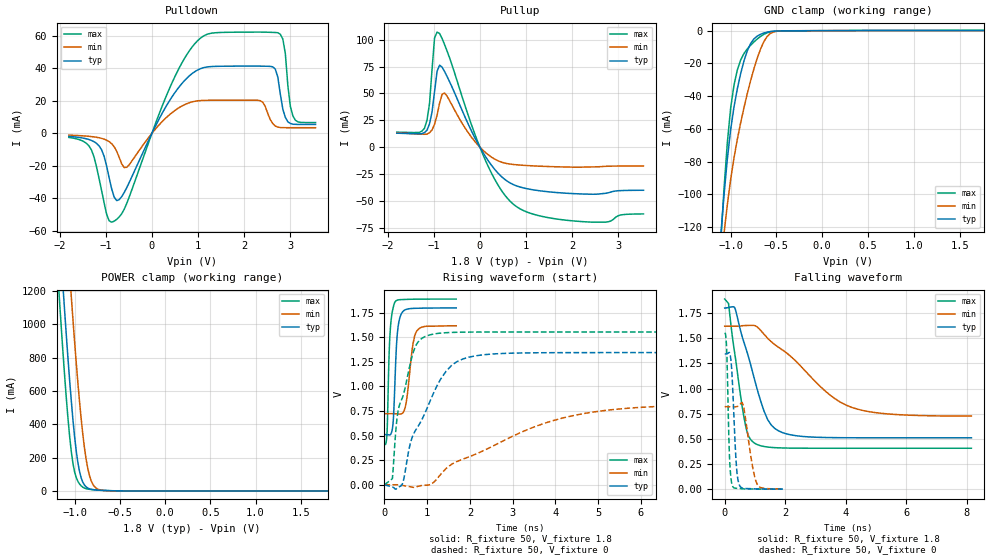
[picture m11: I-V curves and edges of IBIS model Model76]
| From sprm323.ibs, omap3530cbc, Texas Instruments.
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| Model based on original model for BQ0234CS_7LM
|   Sub model BQ0234CS_7LM_PD_ON_1P8
[model]   Model76
|[Input Load]   PD
|[Output Drive]
|Voltage   1.8V
|Mode   I/O
Model_type   I/O
Polarity   Non-Inverting
Enable   Active-Low
Vinl =  0.63
Vinh =  1.17
Cref =  15.0000pF
Rref =  100.0000M
Vref =  0V
Vmeas =  0.9
C_comp   0.8818576p   0.7571797p   1.039848p
[Model Spec]
Vinl   0.63   0.567   0.6615
Vinh   1.17   1.053   1.2285
[Temperature Range]   25   125   -40
[Voltage Range]   1.8   1.62   1.89
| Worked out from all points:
|   slope of the pulldown table from 0 to 0.27 V, typ, clamps not added: 18.2 ohm
|   slope of the pullup table from 0 to 0.27 V, typ, clamps not added: 15.1 ohm
|   GND clamp passes 1 mA (typ) near -0.61 V on its own axis
|   POWER clamp passes 1 mA (typ) near -0.56 V on its own axis
|   rising waveform, R_fixture 50, V_fixture 1.8: 20-80 % time 81.6ps typ, 139ps min, 65.7ps max; typ from 0.51 V to 1.8 V
|   rising waveform, R_fixture 50, V_fixture 0: 20-80 % time 782ps typ, 2.51ns min, 384ps max; typ from 0 V to 1.34 V
|   falling waveform, R_fixture 50, V_fixture 1.8: 20-80 % time 758ps typ, 1.98ns min, 422ps max; typ from 1.8 V to 0.51 V
|   falling waveform, R_fixture 50, V_fixture 0: 20-80 % time 125ps typ, 248ps min, 80ps max; typ from 1.34 V to 0.001 V
[POWER_clamp]
-1.8V     7.03A      7.477A     6.772A
-1.182V   1.672A     2.34A      1.267A
-1.164V   1.518A     2.189A     1.114A
-1.127V   1.216A     1.889A     820.5mA
-1.073V   791.2mA    1.448A     431.2mA
-1.036V   538.2mA    1.164A     234.6mA
-963.6mV  169mA      647.7mA    57.37mA
-909.1mV  52.03mA    338.6mA    22.22mA
-872.7mV  24.23mA    189.8mA    13.46mA
-818.2mV  9.921mA    62.61mA    8.619mA
-709.1mV  3.907mA    5.01mA     3.883mA
1.8V      125.3uA    51.98uA    219uA
[Pulldown]
-1.8V     -1.896mA   -1.14mA    -2.549mA
-1.364V   -3.858mA   -1.868mA   -7.811mA
-1.145V   -7.758mA   -2.749mA   -27.9mA
-818.2mV  -39.37mA   -8.281mA   -54.21mA
-545.5mV  -33.49mA   -20.95mA   -43.25mA
654.5mV   30.89mA    16.9mA     43.68mA
1.418V    41.32mA    20.41mA    62.11mA
2.345V    41.43mA    20.12mA    62.44mA
2.618V    40.99mA    5.968mA    62.24mA
2.782V    24.07mA    3.525mA    61.09mA
3.055V    5.586mA    3.449mA    10.68mA
3.545V    5.467mA    3.446mA    6.63mA
[Pullup]
-1.8V     13mA       13.47mA    13.94mA
-1.2V     13.58mA    11.97mA    17.52mA
-1.091V   21.69mA    13.4mA     40.45mA
-1.036V   32.56mA    16.02mA    72.07mA
-981.8mV  51.55mA    21.35mA    101.5mA
-927.3mV  70.65mA    29.73mA    107.1mA
-818.2mV  74.4mA     49.19mA    101mA
-763.6mV  70.3mA     50.34mA    95.36mA
54.55mV   -4.057mA   -2.362mA   -5.698mA
709.1mV   -34.52mA   -16.04mA   -52.48mA
2.127V    -43.43mA   -18.65mA   -69mA
3.545V    -40.12mA   -17.52mA   -62.13mA
[GND_clamp]
-1.8V     -750.7mA   -623.3mA   -941.3mA
-1.109V   -125.7mA   -143.5mA   -129.9mA
-1.073V   -100.4mA   -123.9mA   -96.51mA
-1.036V   -78.32mA   -106.2mA   -68.27mA
-1V       -60.38mA   -90.77mA   -47.15mA
-963.6mV  -46.54mA   -77.63mA   -33.2mA
-890.9mV  -26.21mA   -56.2mA    -17.88mA
-818.2mV  -12.24mA   -38.36mA   -11.11mA
-709.1mV  -3.293mA   -16.65mA   -5.049mA
-600mV    -851.2uA   -3.412mA   -1.264mA
-490.9mV  -193.3uA   -326.3uA   -232.3uA
1.764V    125uA      52.52uA    217.2uA
[Ramp]
dV/dt_f  0.7809404/0.7631785n  0.5424068/2.010428n   0.9002915/0.426131n
dV/dt_r  0.8335148/0.7828545n  0.5075406/2.539371n   0.9662018/0.3845729n
R_load = 50
[Rising Waveform]
R_fixture = 50
V_fixture = 1.8
V_fixture_min = 1.62
V_fixture_max = 1.89
0s        510.1mV    723.2mV    406.6mV
60ps      510.1mV    723.2mV    520.4mV
104ps     507.5mV    723.3mV    1.259V
136ps     509.4mV    723.6mV    1.572V
202ps     627.8mV    723.9mV    1.796V
242ps     999.6mV    723.1mV    1.854V
300ps     1.53V      720.6mV    1.877V
428ps     1.76V      730.1mV    1.883V
752ps     1.795V     1.56V      1.887V
1.68ns    1.798V     1.616V     1.888V
[Rising Waveform]
R_fixture = 50
V_fixture = 0
V_fixture_min = 0
V_fixture_max = 0
0s        195.2nV    87.26nV    423.3nV
186ps     -22.47mV   203.7uV    62.18mV
308ps     -30.19mV   144.3uV    719.5mV
432ps     23.98mV    -7.241mV   900.4mV
644ps     476.7mV    -23.85mV   1.301V
996ps     777.4mV    -4.058mV   1.515V
1.576ns   1.216V     209.9mV    1.549V
2.236ns   1.317V     330.6mV    1.553V
4.91ns    1.344V     741.2mV    1.553V
9.682ns   1.344V     816.1mV    1.553V
[Falling Waveform]
R_fixture = 50
V_fixture = 1.8
V_fixture_min = 1.62
V_fixture_max = 1.89
0s        1.799V     1.619V     1.888V
126ps     1.804V     1.619V     1.845V
340ps     1.796V     1.619V     1.334V
676ps     1.422V     1.625V     652.2mV
1.008ns   1.066V     1.623V     453.7mV
1.422ns   690mV      1.499V     418.5mV
2.116ns   544.1mV    1.336V     408.2mV
3.386ns   513.2mV    959.2mV    406.7mV
4.186ns   510.8mV    814mV      406.6mV
8.16ns    510.1mV    726.5mV    406.6mV
[Falling Waveform]
R_fixture = 50
V_fixture = 0
V_fixture_min = 0
V_fixture_max = 0
0s        1.344V     819.4mV    1.553V
68ps      1.344V     819.3mV    1.364V
168ps     1.349V     818.5mV    262.1mV
256ps     1.057V     818mV      32.01mV
376ps     278.1mV    818.8mV    8.742mV
492ps     36.54mV    836.9mV    6.364mV
636ps     8.133mV    802.3mV    2.918mV
926ps     4.221mV    215.7mV    1.579mV
1.076ns   2.756mV    48.54mV    1.183mV
1.916ns   1.057mV    3.246mV    221.3uV
